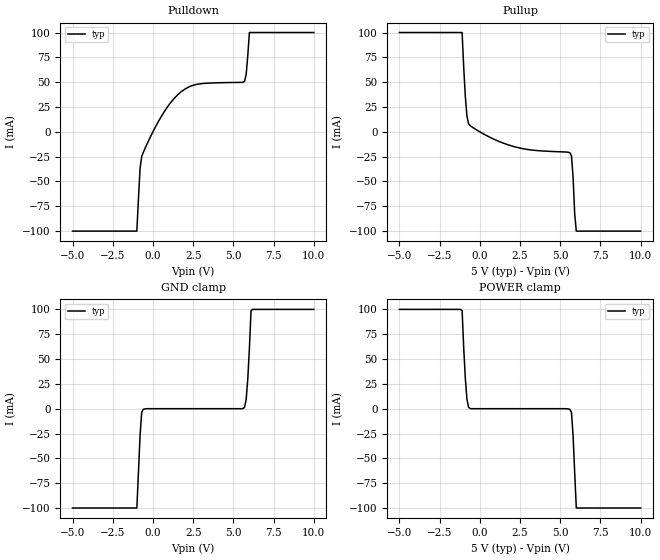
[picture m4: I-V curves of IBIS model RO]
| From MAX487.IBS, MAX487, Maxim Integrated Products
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|   Driver Receiver 3-State Output RO
[Model]   RO
|Signals   R0
Model_type   3-state
Polarity   Non-Inverting
C_comp   0.538pF   NA   NA
[Temperature Range]   25   -40   85
[Voltage Range]   5.00V   4.75V   5.25V
[Pullup Reference]   5.00V   4.75V   5.25V
[Pulldown Reference]   0.00V   0.00V   0.00V
[POWER Clamp Reference]   5.00V   4.75V   5.25V
[GND Clamp Reference]   0.00V   0.00V   0.00V
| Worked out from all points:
|   slope of the pulldown table from 0 to 0.75 V, typ, clamps not added: 35.1 ohm
|   slope of the pullup table from 0 to 0.75 V, typ, clamps not added: 116 ohm
|   GND clamp passes 1 mA (typ) near -0.61 V on its own axis
|   POWER clamp passes 1 mA (typ) near -0.66 V on its own axis
[Pullup]
| Note that the[Pulldown]voltage table is referenced to Vcc
| and is calculated using Vtable=Vcc - Vmeasured.
| Also, the Semiconductor Parameter Analyzer (Force and Sense)
| clamps the supply current to 100mA to protect the system.
| V(V)  I(typ)   I(min)  I(max)
-5V       100mA      NA         NA
-1.1V     100mA      NA         NA
-900mV    35.45mA    NA         NA
-800mV    15.96mA    NA         NA
-600mV    6.201mA    NA         NA
2.2V      -15.2mA    NA         NA
5.6V      -21.06mA   NA         NA
5.7V      -24.07mA   NA         NA
5.8V      -45.57mA   NA         NA
5.9V      -82.46mA   NA         NA
6V        -100mA     NA         NA
10V       -100mA     NA         NA
[Pulldown]
| Note that the[Pulldown]voltage table is referenced to Gnd.
| Also, the Semiconductor Parameter Analyzer (Force and Sense)
| clamps the supply current to 100mA to protect the system.
| V(V)  I(typ)   I(min)  I(max)
-5V       -100mA     NA         NA
-1V       -100mA     NA         NA
-800mV    -36.82mA   NA         NA
-700mV    -24.93mA   NA         NA
400mV     12.11mA    NA         NA
1.3V      33.19mA    NA         NA
2.3V      45.65mA    NA         NA
5.7V      51mA       NA         NA
5.8V      58.1mA     NA         NA
5.9V      77.26mA    NA         NA
6V        100mA      NA         NA
10V       100mA      NA         NA
[POWER_clamp]
| Note that the[POWER_clamp]voltage table is referenced to Vcc
| and is calculated using Vtable=Vcc - Vmeasured.
| Also, the Semiconductor Parameter Analyzer (Force and Sense)
| clamps the supply current to 100mA to protect the system.
| V(V)  I(typ)   I(min)  I(max)
-5V       100mA      NA         NA
-1.1V     98.87mA    NA         NA
-1V       61.12mA    NA         NA
-900mV    30.56mA    NA         NA
-800mV    9.759mA    NA         NA
-700mV    1.504mA    NA         NA
-600mV    109.3uA    NA         NA
5.6V      -651uA     NA         NA
5.7V      -3.944mA   NA         NA
5.8V      -27.01mA   NA         NA
6V        -100mA     NA         NA
10V       -100mA     NA         NA
[GND_clamp]
| Note that the[GND_clamp]voltage table is referenced to Gnd.
| Also, the Semiconductor Parameter Analyzer (Force and Sense)
| clamps the supply current to 100mA to protect the system.
| V(V)  I(typ)   I(min)  I(max)
-5V       -100mA     NA         NA
-1V       -100mA     NA         NA
-800mV    -26.96mA   NA         NA
-700mV    -3.926mA   NA         NA
-600mV    -649.1uA   NA         NA
5.6V      108.8uA    NA         NA
5.7V      1.498mA    NA         NA
5.8V      9.743mA    NA         NA
5.9V      30.53mA    NA         NA
6V        61.1mA     NA         NA
6.1V      98.84mA    NA         NA
10V       100mA      NA         NA
[Ramp]
| variable   typ   min   max
dV/dt_r   3.04/11.9nS   NA   NA
dV/dt_f   3.17/4.85nS   NA   NA
R_load = 5Kohms
|End [Model] RO
